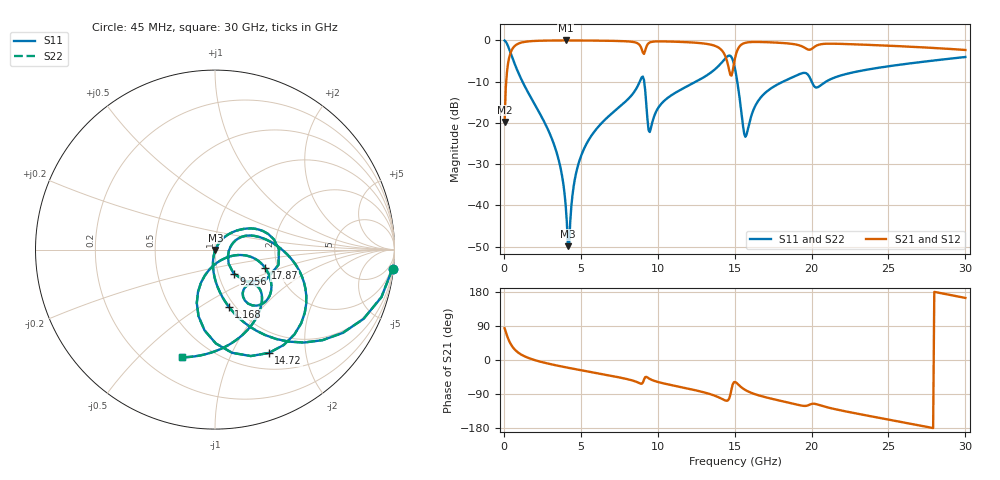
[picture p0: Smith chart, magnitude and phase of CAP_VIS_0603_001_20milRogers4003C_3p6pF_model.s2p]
! S-parameter model data by Modelithics Inc.  support@modelithics.com  813-866-6335  Tampa FL USA
! S-Parameter data specifications:
! Substrate: 20-mil Rogers 4003C, substrate thickness, H=0.508mm, Dielectric constant, Er=3.75
! PCB Mounting Pad Footprint: Pad width, PadW=0.90mm , Pad length, PadL=1.00mm , Pad gap, PadG (edge-to-edge)=1.00mm , Reference planes=3.0mm apart
! Created Wed Nov 18 13:22:03 2015
# hz S ma R 50
! 2 Port Network Data from SP1.SP block
! freq  magS11  angS11  magS21  angS21  magS12  angS12  magS22  angS22
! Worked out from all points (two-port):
!   401 points, 45 MHz to 30 GHz, reference 50 ohm
!   highest |S21| = -0.03 dB at 4.014 GHz (marker M1); lowest = -19.8 dB at 45 MHz (marker M2)
!   |S21| within 3 dB of the highest: 433.1 MHz to 9.05 GHz (8.617 GHz wide, 182 % of centre); 15.12 GHz to end of sweep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
!   lowest |S11| = -49.9 dB at 4.164 GHz (marker M3), VSWR 1.01, Z = 50.2 - j0.265 ohm
!   |S11| at or under -10 dB: 1.206 GHz to 8.829 GHz (7.624 GHz wide, 152 % of centre); 9.118 GHz to 12.49 GHz (3.377 GHz wide, 31.2 % of centre); 15.17 GHz to 18.15 GHz (2.983 GHz wide, 17.9 % of centre)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
!   |S22| runs from -49.9 to 0.0 dB; largest |S21 - S12| = 0
!   S11 on the Smith chart (normalised r, x): 45 MHz: 1, -19; 1.168 GHz: 0.94, -0.67; 9.256 GHz: 1.18, -0.33; 14.72 GHz: 0.70, -1.40; 17.87 GHz: 1.72, -0.38; 30 GHz: 0.34, -0.68
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4.5e7  0.9947 -6.1  0.1025 83.9  0.1025 83.9  0.9947 -6.1
4.194375e8  0.7177 -46.2  0.6957 43.8  0.6957 43.8  0.7177 -46.2
1.168312e9  0.3267 -76.5  0.9437 13.3  0.9437 13.3  0.3267 -76.5
3.265162e9  0.0542 -100.6  0.996 -13.0  0.996 -13.0  0.0542 -100.6
3.714488e9  0.02654 -101.5  0.9969 -16.8  0.9969 -16.8  0.02654 -101.5
4.014038e9  0.01009 -94.6  0.997 -19.3  0.997 -19.3  0.01009 -94.6
4.163812e9  0.003202 -55.5  0.997 -20.5  0.997 -20.5  0.003202 -55.5
5.062462e9  0.04187 58.5  0.9957 -27.4  0.9957 -27.4  0.04187 58.5
8.956612e9  0.3563 0.3  0.7857 -62.7  0.7857 -62.7  0.3563 0.3
9.256162e9  0.1691 -52.1  0.8313 -44.4  0.8313 -44.4  0.1691 -52.1
9.480825e9  0.07746 -5.6  0.9423 -49.9  0.9423 -49.9  0.07746 -5.6
1.007992e10  0.1568 25.7  0.9718 -58.8  0.9718 -58.8  0.1568 25.7
1.344986e10  0.4066 -4.2  0.887 -90.6  0.887 -90.6  0.4066 -4.2
1.434851e10  0.5904 -30.6  0.6712 -106.1  0.6712 -106.1  0.5904 -30.6
1.472295e10  0.6492 -62.5  0.3798 -91.4  0.3798 -91.4  0.6492 -62.5
1.50225e10  0.4539 -97.4  0.6059 -57.8  0.6059 -57.8  0.4539 -97.4
1.569649e10  0.06774 -61.2  0.9339 -79.3  0.9339 -79.3  0.06774 -61.2
1.659514e10  0.1922 -11.0  0.9556 -93.7  0.9556 -93.7  0.1922 -11.0
1.786822e10  0.2974 -20.1  0.9354 -106.6  0.9354 -106.6  0.2974 -20.1
2.003996e10  0.3062 -59.3  0.7954 -115.6  0.7954 -115.6  0.3062 -59.3
2.505742e10  0.4866 -68.9  0.8605 -157.7  0.8605 -157.7  0.4866 -68.9
3e10  0.628 -107.1  0.7643 163.8  0.7643 163.8  0.628 -107.1
